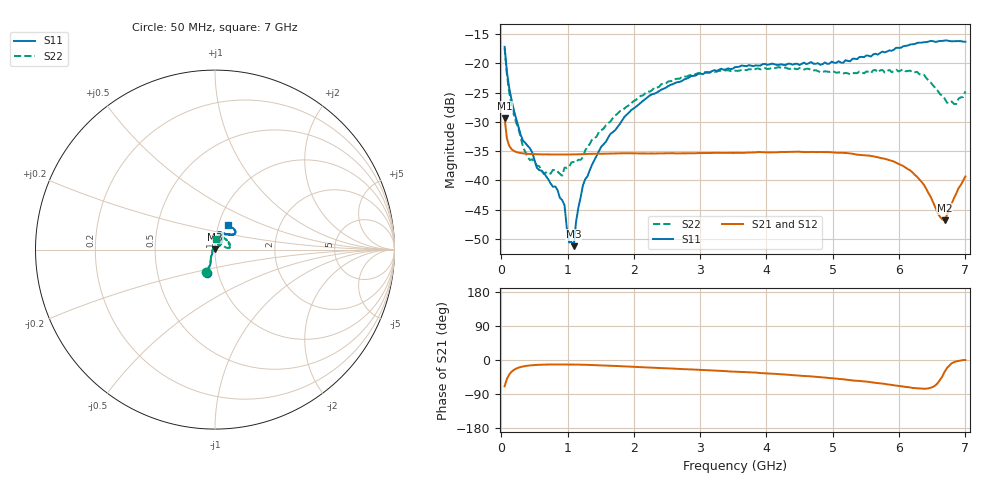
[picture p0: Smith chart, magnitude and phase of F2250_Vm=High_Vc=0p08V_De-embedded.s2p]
! Integrated Device Technology
! Corporate Headquarters
! 6024 Silver Creek Valley Road
! San Jose, CA 95138  USA
! Phone:  1-408-284-8200
! Toll Free:  1-800-223-1366
! Webpage:  http://www.idt.com/
! Timing and RF Division
! 515 Groton Road, Suite 102
! Westford, MA 01886-6024
! Device:  F2250
! Description: Voltage Variable RF Attenuator
! Frequency:  50.0 -  6000.00 MHz
! Package:  3x3 mm Thin QFN Plastic Package: 16 pin
! Ports:  2 RF, 3 DC
!  Pin  1  = GND
!  Pin  2  = NC
!  Pin  3  = RF1  = Port 1
!  Pin  4  = NC
!  Pin  5  = GND
!  Pin  6  = GND
!  Pin  7  = GND
!  Pin  8  = GND
!  Pin  9  = NC
!  Pin 10  = RF2  = Port 2
!  Pin 11  = NC
!  Pin 12  = GND
!  Pin 13  = GND
!  Pin 14  = VCNTRL
!  Pin 15  = VDD
!  Pin 16  = VMODE
! Vcntrl:  0.080 Volts
! Vmode:  +3.300 Volts
! Vdd:  +3.30  Volts
! Current:  1.245 mA
! Data:  The device was measured on a the F2250 evaluation board which has
!  individual transmission lines to the RF pins.  Data was collected
!  using a calibrated network analyzer.  The evaluation board was
!  de-embedded using a TRL calibration technique.
!  The reference plane is the edge of the package pin.
! Misc:  SN 10
!  Action Tracker AT0258
! Date Measured:  2014-11-26
! Date:  2015-10-15  MJV
! Note:
!  Integrated Device Technology supplies this data as a sample of measured
!  data at the package pin for this product.  Your particular data for this
!  product may vary.
!  Data was taken at 25 degrees C.
!  Integrated Device Technology reserves the right to change this data at anytime.
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# GHz S dB R 50
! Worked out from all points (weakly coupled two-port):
!   201 points, 50 MHz to 7 GHz, reference 50 ohm
!   highest |S21| = -29.38 dB at 50 MHz (marker M1); lowest = -46.8 dB at 6.687 GHz (marker M2)
!   lowest |S11| = -51.3 dB at 1.093 GHz (marker M3), VSWR 1.01, Z = 50 + j0.273 ohm
!   |S11| at or under -10 dB: start of sweep to end of sweep
!   |S22| runs from -39.2 to -17.4 dB; largest |S21 - S12| = 6.3e-05
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0.05  -17.18 -108.5  -29.38 -69.5  -29.38 -69.5  -17.37 -110.6
0.08475  -21.47 -107.4  -32.86 -50.1  -32.86 -50.1  -21.87 -109.0
0.15425  -26.23 -116.6  -34.68 -31.0  -34.68 -31.0  -27.11 -120.7
0.29325  -32.27 -127.5  -35.35 -18.4  -35.35 -18.5  -32.66 -133.5
0.3975  -34.11 -142.2  -35.47 -15.0  -35.48 -15.0  -36.07 -158.5
0.5365  -37.87 -154.7  -35.55 -12.9  -35.55 -12.9  -37.49 -179.9
0.64075  -38.75 -162.6  -35.58 -12.2  -35.58 -12.2  -38.90 160.6
0.91875  -43.40 155.9  -35.60 -11.8  -35.60 -11.8  -39.21 127.8
0.9535  -44.26 171.0  -35.60 -11.8  -35.60 -11.8  -37.83 124.2
1.023  -50.64 140.0  -35.59 -11.9  -35.59 -11.9  -37.71 108.1
1.0925  -51.26 89.2  -35.57 -12.0  -35.57 -12.0  -36.85 98.6
1.12725  -47.13 62.3  -35.56 -12.1  -35.56 -12.1  -36.90 91.7
1.2315  -40.85 41.0  -35.52 -12.5  -35.52 -12.5  -36.07 77.3
1.6485  -32.03 41.2  -35.44 -15.2  -35.44 -15.2  -29.92 60.0
2.37825  -24.76 46.7  -35.40 -21.0  -35.39 -21.0  -24.03 53.9
3.525  -20.66 71.7  -35.32 -30.6  -35.32 -30.6  -21.26 73.0
4.7065  -20.06 72.0  -35.15 -43.9  -35.15 -43.9  -21.21 70.3
5.85325  -17.79 40.5  -36.58 -64.9  -36.58 -64.9  -21.13 23.3
6.27025  -16.53 39.4  -39.40 -74.5  -39.40 -74.6  -21.46 8.6
6.68725  -16.11 47.9  -46.82 -31.0  -46.77 -30.7  -26.02 28.4
6.861  -16.21 54.5  -42.31 -3.6  -42.28 -3.6  -26.96 57.4
7  -16.32 62.5  -39.35 -0.1  -39.32 -0.3  -24.82 83.6
